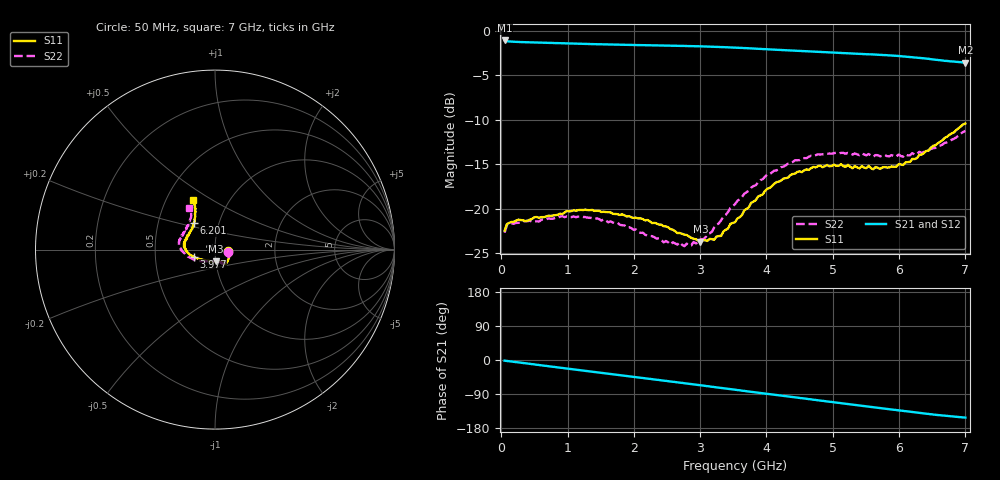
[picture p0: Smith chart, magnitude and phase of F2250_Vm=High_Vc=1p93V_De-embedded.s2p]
! Integrated Device Technology
! Corporate Headquarters
! 6024 Silver Creek Valley Road
! San Jose, CA 95138  USA
! Phone:  1-408-284-8200
! Toll Free:  1-800-223-1366
! Webpage:  http://www.idt.com/
! Timing and RF Division
! 515 Groton Road, Suite 102
! Westford, MA 01886-6024
! Device:  F2250
! Description: Voltage Variable RF Attenuator
! Frequency:  50.0 -  6000.00 MHz
! Package:  3x3 mm Thin QFN Plastic Package: 16 pin
! Ports:  2 RF, 3 DC
!  Pin  1  = GND
!  Pin  2  = NC
!  Pin  3  = RF1  = Port 1
!  Pin  4  = NC
!  Pin  5  = GND
!  Pin  6  = GND
!  Pin  7  = GND
!  Pin  8  = GND
!  Pin  9  = NC
!  Pin 10  = RF2  = Port 2
!  Pin 11  = NC
!  Pin 12  = GND
!  Pin 13  = GND
!  Pin 14  = VCNTRL
!  Pin 15  = VDD
!  Pin 16  = VMODE
! Vcntrl:  1.930 Volts
! Vmode:  +3.300 Volts
! Vdd:  +3.30  Volts
! Current:  1.324 mA
! Data:  The device was measured on a the F2250 evaluation board which has
!  individual transmission lines to the RF pins.  Data was collected
!  using a calibrated network analyzer.  The evaluation board was
!  de-embedded using a TRL calibration technique.
!  The reference plane is the edge of the package pin.
! Misc:  SN 10
!  Action Tracker AT0258
! Date Measured:  2014-11-26
! Date:  2015-10-15  MJV
! Note:
!  Integrated Device Technology supplies this data as a sample of measured
!  data at the package pin for this product.  Your particular data for this
!  product may vary.
!  Data was taken at 25 degrees C.
!  Integrated Device Technology reserves the right to change this data at anytime.
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# GHz S dB R 50
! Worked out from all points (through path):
!   201 points, 50 MHz to 7 GHz, reference 50 ohm
!   highest |S21| = -1.12 dB at 50 MHz (marker M1); lowest = -3.6 dB at 7 GHz (marker M2)
!   group delay of S21, straight-line fit = 61.1 ps
!   lowest |S11| = -23.7 dB at 3.004 GHz (marker M3), VSWR 1.14, Z = 49.9 - j6.54 ohm
!   |S11| at or under -10 dB: start of sweep to end of sweep
!   |S22| runs from -24.2 to -11.3 dB; largest |S21 - S12| = 0.0018
!   S11 on the Smith chart (normalised r, x): 50 MHz: 1.16, -0.02; 3.977 GHz: 0.78, -0.06; 6.201 GHz: 0.76, +0.23; 7 GHz: 0.68, +0.41
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0.05  -22.47 -7.5  -1.12 -1.8  -1.12 -1.8  -22.70 -8.4
0.08475  -21.72 -7.1  -1.20 -2.5  -1.20 -2.5  -21.86 -7.6
0.1195  -21.60 -7.7  -1.23 -3.3  -1.23 -3.3  -21.69 -7.4
0.6755  -20.89 -30.4  -1.37 -15.7  -1.37 -15.7  -21.23 -32.7
1.2315  -20.16 -48.5  -1.49 -27.9  -1.50 -27.9  -20.93 -55.5
1.75275  -20.62 -55.3  -1.59 -39.1  -1.59 -39.1  -21.57 -64.4
2.37825  -21.79 -56.9  -1.68 -52.7  -1.68 -52.7  -23.32 -70.7
2.552  -22.30 -60.8  -1.70 -56.5  -1.70 -56.6  -24.03 -77.2
2.7605  -22.92 -68.3  -1.73 -61.2  -1.74 -61.2  -24.21 -87.7
3.00375  -23.70 -86.9  -1.78 -66.7  -1.78 -66.7  -23.44 -107.3
3.1775  -23.44 -100.7  -1.81 -70.6  -1.82 -70.6  -22.60 -121.2
3.3165  -23.05 -117.9  -1.85 -73.8  -1.85 -73.8  -21.28 -131.4
3.4555  -21.70 -131.1  -1.90 -76.9  -1.90 -76.9  -19.92 -139.9
3.525  -21.53 -135.9  -1.92 -78.5  -1.92 -78.5  -19.50 -143.4
3.97675  -18.02 -162.1  -2.09 -88.6  -2.09 -88.7  -16.42 -164.0
4.4285  -16.08 -175.9  -2.27 -98.6  -2.27 -98.6  -14.58 -178.3
4.7065  -15.31 176.4  -2.37 -104.7  -2.37 -104.7  -14.11 175.6
5.054  -15.19 168.0  -2.50 -112.4  -2.49 -112.5  -13.73 168.1
5.85325  -15.37 141.3  -2.79 -129.9  -2.79 -130.0  -14.12 148.8
6.20075  -14.41 128.6  -3.00 -137.6  -3.00 -137.7  -13.77 139.5
6.54825  -12.88 119.6  -3.27 -144.6  -3.27 -144.7  -13.18 128.1
7  -10.44 113.9  -3.60 -152.0  -3.60 -152.1  -11.27 121.5
